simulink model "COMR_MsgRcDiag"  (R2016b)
settings: Solver=FixedStepDiscrete  StartTime=0.0  StopTime=10.0  FixedStep=0.02  RelTol=1e-3  EnableMultiTasking=on
libraries: simulink x39

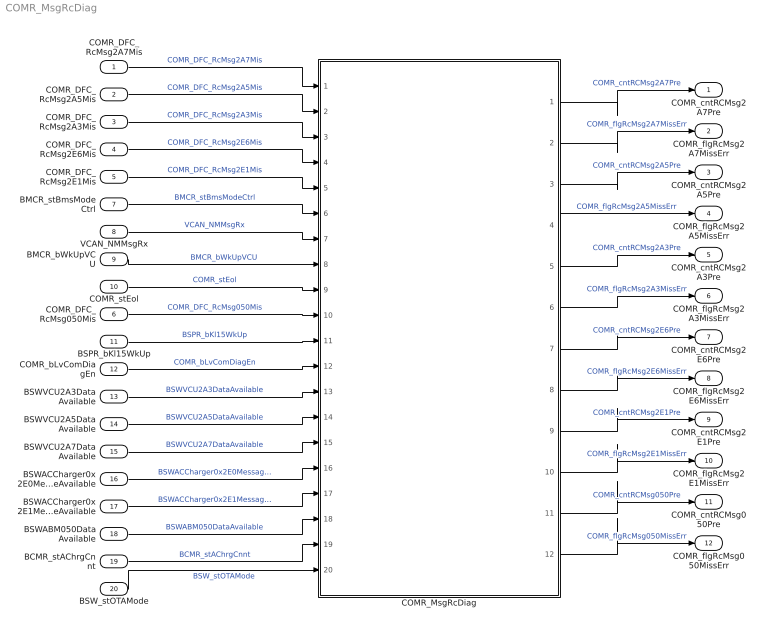
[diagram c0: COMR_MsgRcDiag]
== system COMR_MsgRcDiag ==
  COMR_DFC_RcMsg2A7Mis : Inport
  COMR_DFC_RcMsg2A5Mis : Inport  Port=2
  COMR_DFC_RcMsg2A3Mis : Inport  Port=3
  COMR_DFC_RcMsg2E6Mis : Inport  Port=4
  COMR_DFC_RcMsg2E1Mis : Inport  Port=5
  COMR_DFC_RcMsg050Mis : Inport  Port=6
  BMCR_stBmsModeCtrl : Inport  Port=7  OutDataTypeStr=uint8
  VCAN_NMMsgRx : Inport  Port=8  OutDataTypeStr=boolean
  BMCR_bWkUpVCU : Inport  Port=9  OutDataTypeStr=boolean
  COMR_stEol : Inport  Port=10  OutDataTypeStr=boolean
  BSPR_bKl15WkUp : Inport  Port=11
  COMR_bLvComDiagEn : Inport  Port=12  OutDataTypeStr=boolean
  BSWVCU2A3DataAvailable : Inport  Port=13  OutDataTypeStr=boolean
  BSWVCU2A5DataAvailable : Inport  Port=14  OutDataTypeStr=boolean
  BSWVCU2A7DataAvailable : Inport  Port=15  OutDataTypeStr=boolean
  BSWACCharger0x2E0MessageAvailable : Inport  Port=16
  BSWACCharger0x2E1MessageAvailable : Inport  Port=17  OutDataTypeStr=boolean
  BSWABM050DataAvailable : Inport  Port=18  OutDataTypeStr=boolean
  BCMR_stAChrgCnnt : Inport  Port=19
  BSW_stOTAMode : Inport  Port=20  OutDataTypeStr=boolean
  COMR_MsgRcDiag : Subsystem
  COMR_cntRCMsg2A7Pre : Outport
  COMR_flgRcMsg2A7MissErr : Outport  Port=2
  COMR_cntRCMsg2A5Pre : Outport  Port=3
  COMR_flgRcMsg2A5MissErr : Outport  Port=4
  COMR_cntRCMsg2A3Pre : Outport  Port=5
  COMR_flgRcMsg2A3MissErr : Outport  Port=6
  COMR_cntRCMsg2E6Pre : Outport  Port=7
  COMR_flgRcMsg2E6MissErr : Outport  Port=8
  COMR_cntRCMsg2E1Pre : Outport  Port=9
  COMR_flgRcMsg2E1MissErr : Outport  Port=10
  COMR_cntRCMsg050Pre : Outport  Port=11
  COMR_flgRcMsg050MissErr : Outport  Port=12
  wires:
  COMR_DFC_RcMsg2A7Mis/1 -> COMR_MsgRcDiag/1("COMR_DFC_RcMsg2A7Mis ")  "COMR_DFC_RcMsg2A7Mis"
  COMR_DFC_RcMsg2A5Mis/1 -> COMR_MsgRcDiag/2(COMR_DFC_RcMsg2A5Mis)  "COMR_DFC_RcMsg2A5Mis"
  COMR_DFC_RcMsg2A3Mis/1 -> COMR_MsgRcDiag/3(COMR_DFC_RcMsg2A3Mis)  "COMR_DFC_RcMsg2A3Mis"
  COMR_DFC_RcMsg2E6Mis/1 -> COMR_MsgRcDiag/4(COMR_DFC_RcMsg2E6Mis)  "COMR_DFC_RcMsg2E6Mis"
  COMR_DFC_RcMsg2E1Mis/1 -> COMR_MsgRcDiag/5(COMR_DFC_RcMsg2E1Mis)  "COMR_DFC_RcMsg2E1Mis"
  COMR_DFC_RcMsg050Mis/1 -> COMR_MsgRcDiag/10(COMR_DFC_RcMsg050Mis)  "COMR_DFC_RcMsg050Mis"
  COMR_MsgRcDiag/1(COMR_cntRCMsg2A7Pre) -> COMR_cntRCMsg2A7Pre/1  "COMR_cntRCMsg2A7Pre"
  COMR_MsgRcDiag/2(COMR_flgRcMsg2A7MissErr) -> COMR_flgRcMsg2A7MissErr/1  "COMR_flgRcMsg2A7MissErr"
  COMR_MsgRcDiag/3(COMR_cntRCMsg2A5Pre) -> COMR_cntRCMsg2A5Pre/1  "COMR_cntRCMsg2A5Pre"
  COMR_MsgRcDiag/4(COMR_flgRcMsg2A5MissErr) -> COMR_flgRcMsg2A5MissErr/1  "COMR_flgRcMsg2A5MissErr"
  COMR_MsgRcDiag/5(COMR_cntRCMsg2A3Pre) -> COMR_cntRCMsg2A3Pre/1  "COMR_cntRCMsg2A3Pre"
  COMR_MsgRcDiag/6(COMR_flgRcMsg2A3MissErr) -> COMR_flgRcMsg2A3MissErr/1  "COMR_flgRcMsg2A3MissErr"
  COMR_MsgRcDiag/7(COMR_cntRCMsg2E6Pre) -> COMR_cntRCMsg2E6Pre/1  "COMR_cntRCMsg2E6Pre"
  COMR_MsgRcDiag/8(COMR_flgRcMsg2E6MissErr) -> COMR_flgRcMsg2E6MissErr/1  "COMR_flgRcMsg2E6MissErr"
  COMR_MsgRcDiag/9(COMR_cntRCMsg2E1Pre) -> COMR_cntRCMsg2E1Pre/1  "COMR_cntRCMsg2E1Pre"
  COMR_MsgRcDiag/10(COMR_flgRcMsg2E1MissErr) -> COMR_flgRcMsg2E1MissErr/1  "COMR_flgRcMsg2E1MissErr"
  COMR_MsgRcDiag/12(COMR_flgRcMsg050MissErr) -> COMR_flgRcMsg050MissErr/1  "COMR_flgRcMsg050MissErr"
  BMCR_stBmsModeCtrl/1 -> COMR_MsgRcDiag/6(BMCR_stBmsModeCtrl)  "BMCR_stBmsModeCtrl"
  COMR_MsgRcDiag/11(COMR_cntRCMsg050Pre) -> COMR_cntRCMsg050Pre/1  "COMR_cntRCMsg050Pre"
  VCAN_NMMsgRx/1 -> COMR_MsgRcDiag/7(VCAN_NMMsgRx)  "VCAN_NMMsgRx"
  BMCR_bWkUpVCU/1 -> COMR_MsgRcDiag/8(BMCR_bWkUpVCU)  "BMCR_bWkUpVCU"
  COMR_stEol/1 -> COMR_MsgRcDiag/9(COMR_stEol)  "COMR_stEol"
  BSPR_bKl15WkUp/1 -> COMR_MsgRcDiag/11(BSPR_bKl15WkUp)  "BSPR_bKl15WkUp"
  COMR_bLvComDiagEn/1 -> COMR_MsgRcDiag/12(COMR_bLvComDiagEn)  "COMR_bLvComDiagEn"
  BSWVCU2A3DataAvailable/1 -> COMR_MsgRcDiag/13(BSWVCU2A3DataAvailable)  "BSWVCU2A3DataAvailable"
  BSWVCU2A5DataAvailable/1 -> COMR_MsgRcDiag/14(BSWVCU2A5DataAvailable)  "BSWVCU2A5DataAvailable"
  BSWVCU2A7DataAvailable/1 -> COMR_MsgRcDiag/15(BSWVCU2A7DataAvailable)  "BSWVCU2A7DataAvailable"
  BSWACCharger0x2E0MessageAvailable/1 -> COMR_MsgRcDiag/16(BSWACCharger0x2E0MessageAvailable)  "BSWACCharger0x2E0MessageAvailable"
  BSWACCharger0x2E1MessageAvailable/1 -> COMR_MsgRcDiag/17(BSWACCharger0x2E1MessageAvailable)  "BSWACCharger0x2E1MessageAvailable"
  BSWABM050DataAvailable/1 -> COMR_MsgRcDiag/18(BSWABM050DataAvailable)  "BSWABM050DataAvailable"
  BCMR_stAChrgCnnt/1 -> COMR_MsgRcDiag/19(BCMR_stAChrgCnnt)  "BCMR_stAChrgCnnt"
  BSW_stOTAMode/1 -> COMR_MsgRcDiag/20(BSW_stOTAMode)  "BSW_stOTAMode"

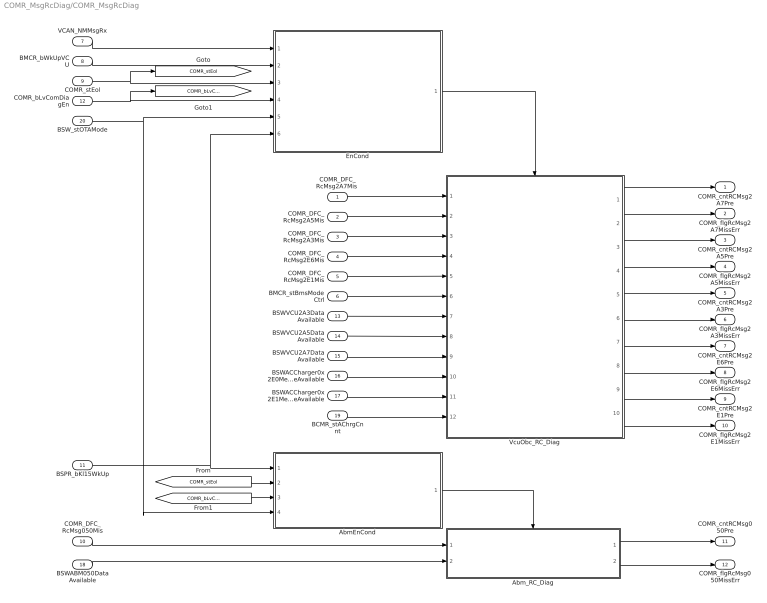
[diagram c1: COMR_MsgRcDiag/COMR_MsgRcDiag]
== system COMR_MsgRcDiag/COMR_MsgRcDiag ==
  "COMR_DFC_RcMsg2A7Mis " : Inport
  COMR_DFC_RcMsg2A5Mis : Inport  Port=2
  COMR_DFC_RcMsg2A3Mis : Inport  Port=3
  COMR_DFC_RcMsg2E6Mis : Inport  Port=4
  COMR_DFC_RcMsg2E1Mis : Inport  Port=5
  BMCR_stBmsModeCtrl : Inport  Port=6
  VCAN_NMMsgRx : Inport  Port=7  OutDataTypeStr=boolean
  BMCR_bWkUpVCU : Inport  Port=8  OutDataTypeStr=boolean
  COMR_stEol : Inport  Port=9  OutDataTypeStr=boolean
  COMR_DFC_RcMsg050Mis : Inport  Port=10
  BSPR_bKl15WkUp : Inport  Port=11  OutDataTypeStr=boolean
  COMR_bLvComDiagEn : Inport  Port=12  OutDataTypeStr=boolean
  BSWVCU2A3DataAvailable : Inport  Port=13  OutDataTypeStr=boolean
  BSWVCU2A5DataAvailable : Inport  Port=14  OutDataTypeStr=boolean
  BSWVCU2A7DataAvailable : Inport  Port=15  OutDataTypeStr=boolean
  BSWACCharger0x2E0MessageAvailable : Inport  Port=16
  BSWACCharger0x2E1MessageAvailable : Inport  Port=17  OutDataTypeStr=boolean
  BSWABM050DataAvailable : Inport  Port=18  OutDataTypeStr=boolean
  BCMR_stAChrgCnnt : Inport  Port=19
  BSW_stOTAMode : Inport  Port=20  OutDataTypeStr=boolean
  AbmEnCond : Subsystem
  Abm_RC_Diag : Subsystem
  EnCond : Subsystem
  VcuObc_RC_Diag : Subsystem
  COMR_cntRCMsg2A7Pre : Outport
  COMR_flgRcMsg2A7MissErr : Outport  Port=2
  COMR_cntRCMsg2A5Pre : Outport  Port=3
  COMR_flgRcMsg2A5MissErr : Outport  Port=4
  COMR_cntRCMsg2A3Pre : Outport  Port=5
  COMR_flgRcMsg2A3MissErr : Outport  Port=6
  COMR_cntRCMsg2E6Pre : Outport  Port=7
  COMR_flgRcMsg2E6MissErr : Outport  Port=8
  COMR_cntRCMsg2E1Pre : Outport  Port=9
  COMR_flgRcMsg2E1MissErr : Outport  Port=10
  COMR_cntRCMsg050Pre : Outport  Port=11
  COMR_flgRcMsg050MissErr : Outport  Port=12
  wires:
  VCAN_NMMsgRx/1 -> EnCond/1(VCAN_NMMsgRx)
  BMCR_bWkUpVCU/1 -> EnCond/2(BMCR_bWkUpVCU)
  COMR_stEol/1 -> EnCond/3(COMR_stEol), [COMR_stEol]
  "COMR_DFC_RcMsg2A7Mis "/1 -> VcuObc_RC_Diag/1(COMR_DFC_RcMsg2A7Mis)
  COMR_DFC_RcMsg2A5Mis/1 -> VcuObc_RC_Diag/2(COMR_DFC_RcMsg2A5Mis)
  COMR_DFC_RcMsg2A3Mis/1 -> VcuObc_RC_Diag/3(COMR_DFC_RcMsg2A3Mis)
  COMR_DFC_RcMsg2E6Mis/1 -> VcuObc_RC_Diag/4(COMR_DFC_RcMsg2E6Mis)
  COMR_DFC_RcMsg2E1Mis/1 -> VcuObc_RC_Diag/5(COMR_DFC_RcMsg2E1Mis)
  BMCR_stBmsModeCtrl/1 -> VcuObc_RC_Diag/6(BMCR_stBmsModeCtrl)
  VcuObc_RC_Diag/1(COMR_cntRCMsg2A7Pre) -> COMR_cntRCMsg2A7Pre/1
  VcuObc_RC_Diag/2(COMR_flgRcMsg2A7MissErr) -> COMR_flgRcMsg2A7MissErr/1
  VcuObc_RC_Diag/3(COMR_cntRCMsg2A5Pre) -> COMR_cntRCMsg2A5Pre/1
  VcuObc_RC_Diag/4(COMR_flgRcMsg2A5MissErr) -> COMR_flgRcMsg2A5MissErr/1
  VcuObc_RC_Diag/5(COMR_cntRCMsg2A3Pre) -> COMR_cntRCMsg2A3Pre/1
  VcuObc_RC_Diag/6(COMR_flgRcMsg2A3MissErr) -> COMR_flgRcMsg2A3MissErr/1
  VcuObc_RC_Diag/7(COMR_cntRCMsg2E6Pre) -> COMR_cntRCMsg2E6Pre/1
  VcuObc_RC_Diag/8(COMR_flgRcMsg2E6MissErr) -> COMR_flgRcMsg2E6MissErr/1
  VcuObc_RC_Diag/9(COMR_cntRCMsg2E1Pre) -> COMR_cntRCMsg2E1Pre/1
  VcuObc_RC_Diag/10(COMR_flgRcMsg2E1MissErr) -> COMR_flgRcMsg2E1MissErr/1
  EnCond/1(COMR_bMsgRcDiagEn) -> VcuObc_RC_Diag/Enable
  COMR_DFC_RcMsg050Mis/1 -> Abm_RC_Diag/1(COMR_DFC_RcMsg050Mis)
  Abm_RC_Diag/1(COMR_cntRCMsg050Pre) -> COMR_cntRCMsg050Pre/1
  Abm_RC_Diag/2(COMR_flgRcMsg050MissErr) -> COMR_flgRcMsg050MissErr/1
  AbmEnCond/1(COMR_bAbmRcDiagEn) -> Abm_RC_Diag/Enable
  BSPR_bKl15WkUp/1 -> EnCond/6(BSPR_bKl15WkUp), AbmEnCond/1(BSPR_bKl15WkUp)
  [COMR_stEol] -> AbmEnCond/2(COMR_stEol)
  COMR_bLvComDiagEn/1 -> EnCond/4(COMR_bLvComDiagEn), [COMR_bLvComDiagEn]
  [COMR_bLvComDiagEn] -> AbmEnCond/3(COMR_bLvComDiagEn)
  BSWACCharger0x2E1MessageAvailable/1 -> VcuObc_RC_Diag/11(BSWACCharger0x2E1MessageAvailable)
  BSWACCharger0x2E0MessageAvailable/1 -> VcuObc_RC_Diag/10(BSWACCharger0x2E0MessageAvailable)
  BSWVCU2A7DataAvailable/1 -> VcuObc_RC_Diag/9(BSWVCU2A7DataAvailable)
  BSWVCU2A5DataAvailable/1 -> VcuObc_RC_Diag/8(BSWVCU2A5DataAvailable)
  BSWVCU2A3DataAvailable/1 -> VcuObc_RC_Diag/7(BSWVCU2A3DataAvailable)
  BSWABM050DataAvailable/1 -> Abm_RC_Diag/2(BSWABM050DataAvailable)
  BCMR_stAChrgCnnt/1 -> VcuObc_RC_Diag/12(BCMR_stAChrgCnnt)
  BSW_stOTAMode/1 -> AbmEnCond/4(BSW_stOTAMode), EnCond/5(BSW_stOTAMode)

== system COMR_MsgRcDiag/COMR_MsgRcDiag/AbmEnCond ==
  BSPR_bKl15WkUp : Inport  OutDataTypeStr=boolean
  COMR_stEol : Inport  Port=2  OutDataTypeStr=boolean
  COMR_bLvComDiagEn : Inport  Port=3  OutDataTypeStr=boolean
  BSW_stOTAMode : Inport  Port=4  OutDataTypeStr=boolean
  Constant1 : Constant  Value=2  OutDataTypeStr=single
  Logical Operator1 : Logic  AllPortsSameDT=off  OutDataTypeStr=boolean
  Logical Operator2 : Logic  Operator=NOT  AllPortsSameDT=off  OutDataTypeStr=boolean
  Logical Operator3 : Logic  Inputs=3  AllPortsSameDT=off  OutDataTypeStr=boolean
  Logical Operator4 : Logic  Operator=NOT  AllPortsSameDT=off  OutDataTypeStr=boolean
  TONV_10msTimeDebounce : Subsystem  TreatAsAtomicUnit=on  RTWFcnName=TONV_10msTimeDebounce  RTWFileName=SrvLib
  COMR_bAbmRcDiagEn : Outport
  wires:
  Logical Operator2/1 -> Logical Operator1/2
  COMR_stEol/1 -> Logical Operator2/1
  BSPR_bKl15WkUp/1 -> Logical Operator1/1
  Logical Operator3/1 -> COMR_bAbmRcDiagEn/1  "COMR_bAbmRcDiagEn"
  Constant1/1 -> TONV_10msTimeDebounce/2(T)
  Logical Operator1/1 -> TONV_10msTimeDebounce/1(u)
  COMR_bLvComDiagEn/1 -> Logical Operator3/2
  TONV_10msTimeDebounce/1(y) -> Logical Operator3/1
  BSW_stOTAMode/1 -> Logical Operator4/1
  Logical Operator4/1 -> Logical Operator3/3

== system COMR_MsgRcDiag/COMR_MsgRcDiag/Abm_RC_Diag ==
  COMR_DFC_RcMsg050Mis : Inport
  BSWABM050DataAvailable : Inport  Port=2  OutDataTypeStr=boolean
  Enable : EnablePort  StatesWhenEnabling=reset
  Constant : Constant  Value=0  OutDataTypeStr=uint8
  DSM_ReportCheck : Subsystem  TreatAsAtomicUnit=on  RTWFcnName=DSM_ReportCheck  RTWFileName=SrvLib
  Data Store Read3 : DataStoreRead  DataStoreName=DFC_RcMsg050Mis
  Data Store Write3 : DataStoreWrite  DataStoreName=DFC_RcMsg050Mis
  Logical Operator2 : Logic  Operator=NOT  AllPortsSameDT=off  OutDataTypeStr=boolean
  Terminator : Terminator
  COMR_cntRCMsg050Pre : Outport
  COMR_flgRcMsg050MissErr : Outport  Port=2
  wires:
  COMR_DFC_RcMsg050Mis/1 -> COMR_flgRcMsg050MissErr/1, DSM_ReportCheck/2(Err), Logical Operator2/1
  DSM_ReportCheck/1(Dfc_id) -> Data Store Write3/1
  Constant/1 -> COMR_cntRCMsg050Pre/1
  Data Store Read3/1 -> DSM_ReportCheck/1(Dfc_id_nv)
  Logical Operator2/1 -> DSM_ReportCheck/3(Heal)
  BSWABM050DataAvailable/1 -> Terminator/1

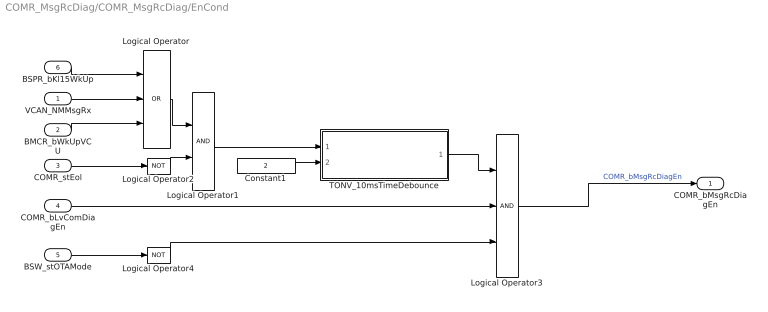
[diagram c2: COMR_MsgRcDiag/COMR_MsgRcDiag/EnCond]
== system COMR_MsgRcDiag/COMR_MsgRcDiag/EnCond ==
  VCAN_NMMsgRx : Inport  OutDataTypeStr=boolean
  BMCR_bWkUpVCU : Inport  Port=2  OutDataTypeStr=boolean
  COMR_stEol : Inport  Port=3  OutDataTypeStr=boolean
  COMR_bLvComDiagEn : Inport  Port=4  OutDataTypeStr=boolean
  BSW_stOTAMode : Inport  Port=5  OutDataTypeStr=boolean
  BSPR_bKl15WkUp : Inport  Port=6  OutDataTypeStr=boolean
  Constant1 : Constant  Value=2  OutDataTypeStr=single
  Logical Operator : Logic  Operator=OR  Inputs=3  AllPortsSameDT=off  OutDataTypeStr=boolean
  Logical Operator1 : Logic  AllPortsSameDT=off  OutDataTypeStr=boolean
  Logical Operator2 : Logic  Operator=NOT  AllPortsSameDT=off  OutDataTypeStr=boolean
  Logical Operator3 : Logic  Inputs=3  AllPortsSameDT=off  OutDataTypeStr=boolean
  Logical Operator4 : Logic  Operator=NOT  AllPortsSameDT=off  OutDataTypeStr=boolean
  TONV_10msTimeDebounce : Subsystem  TreatAsAtomicUnit=on  RTWFcnName=TONV_10msTimeDebounce  RTWFileName=SrvLib
  COMR_bMsgRcDiagEn : Outport
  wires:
  Logical Operator1/1 -> TONV_10msTimeDebounce/1(u)
  Constant1/1 -> TONV_10msTimeDebounce/2(T)
  Logical Operator3/1 -> COMR_bMsgRcDiagEn/1  "COMR_bMsgRcDiagEn"
  Logical Operator/1 -> Logical Operator1/1
  COMR_stEol/1 -> Logical Operator2/1
  Logical Operator2/1 -> Logical Operator1/2
  TONV_10msTimeDebounce/1(y) -> Logical Operator3/1
  COMR_bLvComDiagEn/1 -> Logical Operator3/2
  VCAN_NMMsgRx/1 -> Logical Operator/2
  BMCR_bWkUpVCU/1 -> Logical Operator/3
  BSPR_bKl15WkUp/1 -> Logical Operator/1
  BSW_stOTAMode/1 -> Logical Operator4/1
  Logical Operator4/1 -> Logical Operator3/3

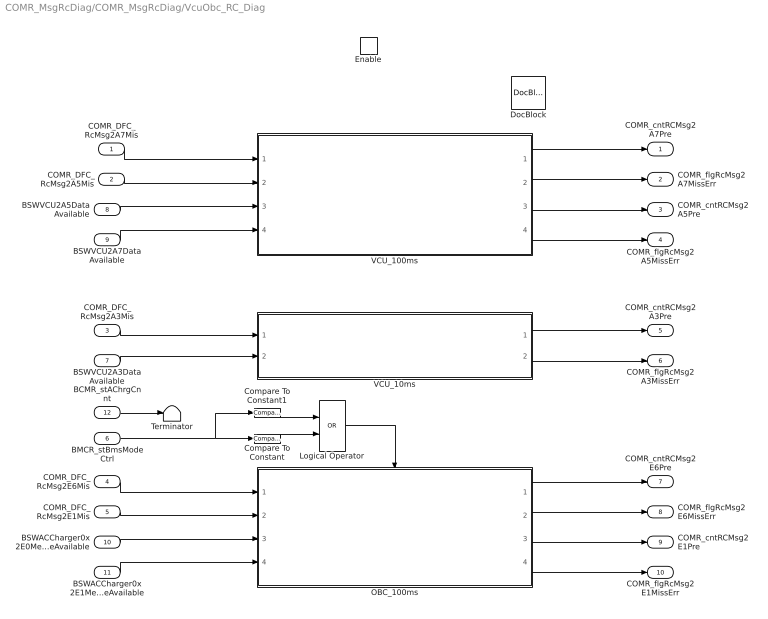
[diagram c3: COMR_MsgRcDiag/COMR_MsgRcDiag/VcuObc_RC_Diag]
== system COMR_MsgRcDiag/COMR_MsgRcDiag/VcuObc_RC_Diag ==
  COMR_DFC_RcMsg2A7Mis : Inport
  COMR_DFC_RcMsg2A5Mis : Inport  Port=2
  COMR_DFC_RcMsg2A3Mis : Inport  Port=3
  COMR_DFC_RcMsg2E6Mis : Inport  Port=4
  COMR_DFC_RcMsg2E1Mis : Inport  Port=5
  BMCR_stBmsModeCtrl : Inport  Port=6
  BSWVCU2A3DataAvailable : Inport  Port=7  OutDataTypeStr=boolean
  BSWVCU2A5DataAvailable : Inport  Port=8  OutDataTypeStr=boolean
  BSWVCU2A7DataAvailable : Inport  Port=9  OutDataTypeStr=boolean
  BSWACCharger0x2E0MessageAvailable : Inport  Port=10
  BSWACCharger0x2E1MessageAvailable : Inport  Port=11  OutDataTypeStr=boolean
  BCMR_stAChrgCnnt : Inport  Port=12
  Enable : EnablePort  StatesWhenEnabling=reset
  Compare To Constant : simulink/Logic and Bit Operations/Compare To Constant  relop===  const=6  OutDataTypeStr=boolean
  Compare To Constant1 : simulink/Logic and Bit Operations/Compare To Constant  relop===  const=11  OutDataTypeStr=boolean
  DocBlock : simulink/Model-Wide Utilities/DocBlock  DocumentType=Text
  Logical Operator : Logic  Operator=OR  AllPortsSameDT=off  OutDataTypeStr=boolean
  OBC_100ms : Subsystem
  Terminator : Terminator
  VCU_100ms : Subsystem
  VCU_10ms : Subsystem
  COMR_cntRCMsg2A7Pre : Outport  InitialOutput=[0]
  COMR_flgRcMsg2A7MissErr : Outport  Port=2  InitialOutput=[0]
  COMR_cntRCMsg2A5Pre : Outport  Port=3  InitialOutput=[0]
  COMR_flgRcMsg2A5MissErr : Outport  Port=4  InitialOutput=[0]
  COMR_cntRCMsg2A3Pre : Outport  Port=5
  COMR_flgRcMsg2A3MissErr : Outport  Port=6
  COMR_cntRCMsg2E6Pre : Outport  Port=7  InitialOutput=[0]
  COMR_flgRcMsg2E6MissErr : Outport  Port=8  InitialOutput=[0]
  COMR_cntRCMsg2E1Pre : Outport  Port=9  InitialOutput=[0]
  COMR_flgRcMsg2E1MissErr : Outport  Port=10  InitialOutput=[0]
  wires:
  COMR_DFC_RcMsg2E6Mis/1 -> OBC_100ms/1(COMR_DFC_RcMsg2E6Mis)
  COMR_DFC_RcMsg2E1Mis/1 -> OBC_100ms/2(COMR_DFC_RcMsg2E1Mis)
  OBC_100ms/1(COMR_cntRCMsg2E6Pre) -> COMR_cntRCMsg2E6Pre/1
  OBC_100ms/2(COMR_flgRcMsg2E6MissErr) -> COMR_flgRcMsg2E6MissErr/1
  OBC_100ms/3(COMR_cntRCMsg2E1Pre) -> COMR_cntRCMsg2E1Pre/1
  OBC_100ms/4(COMR_flgRcMsg2E1MissErr) -> COMR_flgRcMsg2E1MissErr/1
  BMCR_stBmsModeCtrl/1 -> Compare To Constant1/1, Compare To Constant/1
  COMR_DFC_RcMsg2A7Mis/1 -> VCU_100ms/1(COMR_DFC_RcMsg2A7Mis)
  COMR_DFC_RcMsg2A5Mis/1 -> VCU_100ms/2(COMR_DFC_RcMsg2A5Mis)
  VCU_100ms/1(COMR_cntRCMsg2A7Pre) -> COMR_cntRCMsg2A7Pre/1
  VCU_100ms/2(COMR_flgRcMsg2A7MissErr) -> COMR_flgRcMsg2A7MissErr/1
  VCU_100ms/3(COMR_cntRCMsg2A5Pre) -> COMR_cntRCMsg2A5Pre/1
  VCU_100ms/4(COMR_flgRcMsg2A5MissErr) -> COMR_flgRcMsg2A5MissErr/1
  COMR_DFC_RcMsg2A3Mis/1 -> VCU_10ms/1(COMR_DFC_RcMsg2A3Mis)
  VCU_10ms/1(COMR_cntRCMsg2A3Pre) -> COMR_cntRCMsg2A3Pre/1
  VCU_10ms/2(COMR_flgRcMsg2A3MissErr) -> COMR_flgRcMsg2A3MissErr/1
  BSWVCU2A5DataAvailable/1 -> VCU_100ms/3(BSWVCU2A5DataAvailable)
  BSWVCU2A7DataAvailable/1 -> VCU_100ms/4(BSWVCU2A7DataAvailable)
  BSWVCU2A3DataAvailable/1 -> VCU_10ms/2(BSWVCU2A3DataAvailable)
  BSWACCharger0x2E0MessageAvailable/1 -> OBC_100ms/3(BSWACCharger0x2E0MessageAvailable)
  BSWACCharger0x2E1MessageAvailable/1 -> OBC_100ms/4(BSWACCharger0x2E1MessageAvailable)
  Compare To Constant1/1 -> Logical Operator/1
  Compare To Constant/1 -> Logical Operator/2
  Logical Operator/1 -> OBC_100ms/Enable
  BCMR_stAChrgCnnt/1 -> Terminator/1

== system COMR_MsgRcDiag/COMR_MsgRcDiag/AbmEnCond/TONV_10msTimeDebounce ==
  note: Turn On Delay Time Deboune
  u : Inport
  T : Inport  Port=2
  Add : Sum
  Constant1 : Constant  Value=0  OutDataTypeStr=single
  Constant2 : Constant  OutDataTypeStr=uint8
  Constant3 : Constant  Value=0  OutDataTypeStr=uint8
  Constant4 : Constant  Value=0.01  OutDataTypeStr=single
  Delay : Delay  DelayLength=1  InitialCondition=0
  MinMax : MinMax  Inputs=2
  Product : Product  OutMin=[0]  OutMax=[65535]  OutDataTypeStr=single
  Relational Operator : RelationalOperator  Operator=>  OutDataTypeStr=boolean  RndMeth=Simplest
  Switch : Switch  Criteria=u2 ~= 0
  Switch1 : Switch  Criteria=u2 ~= 0
  y : Outport
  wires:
  Switch1/1 -> Product/1
  Constant3/1 -> Switch1/3
  Constant2/1 -> Switch1/1
  u/1 -> Switch1/2, Switch/2
  Constant4/1 -> Switch/1
  Constant1/1 -> Switch/3
  Add/1 -> Product/2
  Product/1 -> Relational Operator/1, Delay/1
  Switch/1 -> Add/1
  Delay/1 -> MinMax/2
  Relational Operator/1 -> y/1
  T/1 -> MinMax/1, Relational Operator/2
  MinMax/1 -> Add/2

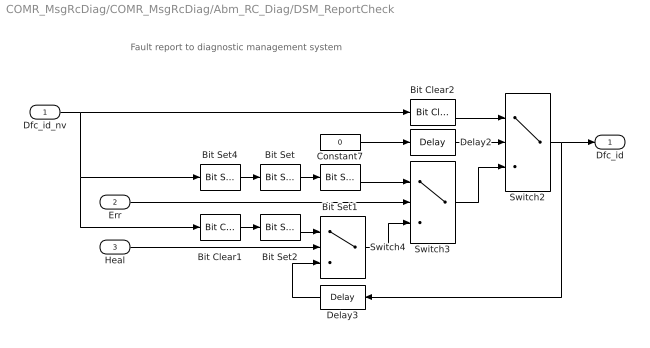
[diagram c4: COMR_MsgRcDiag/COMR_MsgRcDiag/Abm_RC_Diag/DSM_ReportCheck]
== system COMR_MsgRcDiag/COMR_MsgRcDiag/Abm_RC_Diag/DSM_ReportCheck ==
  note: Fault report to diagnostic management system
  Dfc_id_nv : Inport  OutDataTypeStr=uint8
  Err : Inport  Port=2
  Heal : Inport  Port=3
  Bit Clear1 : simulink/Logic and Bit Operations/Bit Clear  iBit=4
  Bit Clear2 : simulink/Logic and Bit Operations/Bit Clear  iBit=3
  Bit Set : simulink/Logic and Bit Operations/Bit Set  iBit=4
  Bit Set1 : simulink/Logic and Bit Operations/Bit Set  iBit=3
  Bit Set2 : simulink/Logic and Bit Operations/Bit Set  iBit=3
  Bit Set4 : simulink/Logic and Bit Operations/Bit Set  iBit=7
  Constant7 : Constant  Value=0  OutDataTypeStr=boolean
  Delay2 : Delay  DelayLength=1  InitialCondition=1
  Delay3 : Delay  DelayLength=1  InitialCondition=0
  Switch2 : Switch  Criteria=u2 ~= 0
  Switch3 : Switch  Criteria=u2 ~= 0
  Switch4 : Switch  Criteria=u2 ~= 0
  Dfc_id : Outport  OutDataTypeStr=uint8
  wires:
  Dfc_id_nv/1 -> Bit Clear2/1, Bit Set4/1, Bit Clear1/1
  Bit Set4/1 -> Bit Set/1
  Constant7/1 -> Delay2/1
  Delay2/1 -> Switch2/2
  Switch3/1 -> Switch2/3
  Bit Clear2/1 -> Switch2/1
  Switch2/1 -> Delay3/1, Dfc_id/1
  Bit Set1/1 -> Switch3/1
  Bit Set/1 -> Bit Set1/1
  Switch4/1 -> Switch3/3
  Err/1 -> Switch3/2
  Bit Set2/1 -> Switch4/1
  Bit Clear1/1 -> Bit Set2/1
  Delay3/1 -> Switch4/3
  Heal/1 -> Switch4/2

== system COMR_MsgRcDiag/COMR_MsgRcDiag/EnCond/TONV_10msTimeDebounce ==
  note: Turn On Delay Time Deboune
  u : Inport
  T : Inport  Port=2
  Add : Sum
  Constant1 : Constant  Value=0  OutDataTypeStr=single
  Constant2 : Constant  OutDataTypeStr=uint8
  Constant3 : Constant  Value=0  OutDataTypeStr=uint8
  Constant4 : Constant  Value=0.01  OutDataTypeStr=single
  Delay : Delay  DelayLength=1  InitialCondition=0
  MinMax : MinMax  Inputs=2
  Product : Product  OutMin=[0]  OutMax=[65535]  OutDataTypeStr=single
  Relational Operator : RelationalOperator  Operator=>  OutDataTypeStr=boolean  RndMeth=Simplest
  Switch : Switch  Criteria=u2 ~= 0
  Switch1 : Switch  Criteria=u2 ~= 0
  y : Outport
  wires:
  MinMax/1 -> Add/2
  T/1 -> Relational Operator/2, MinMax/1
  Relational Operator/1 -> y/1
  Delay/1 -> MinMax/2
  Switch/1 -> Add/1
  Product/1 -> Delay/1, Relational Operator/1
  Add/1 -> Product/2
  Constant1/1 -> Switch/3
  Constant4/1 -> Switch/1
  u/1 -> Switch/2, Switch1/2
  Constant2/1 -> Switch1/1
  Constant3/1 -> Switch1/3
  Switch1/1 -> Product/1

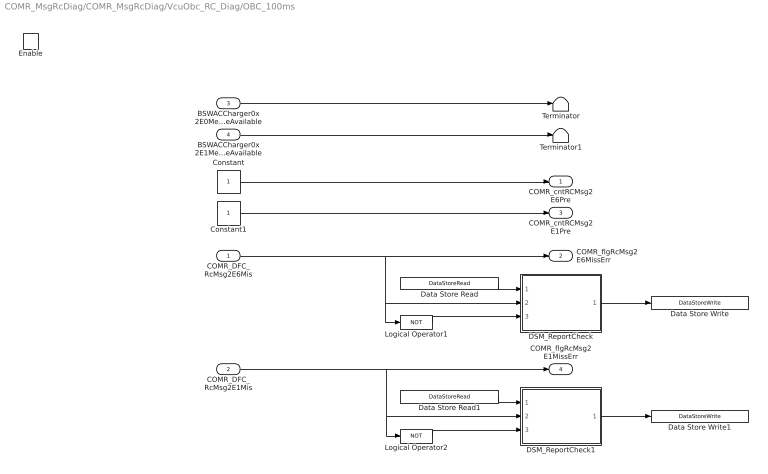
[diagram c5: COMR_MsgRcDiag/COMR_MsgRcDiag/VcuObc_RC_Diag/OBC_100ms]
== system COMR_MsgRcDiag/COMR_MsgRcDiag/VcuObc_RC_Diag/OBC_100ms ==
  COMR_DFC_RcMsg2E6Mis : Inport
  COMR_DFC_RcMsg2E1Mis : Inport  Port=2
  BSWACCharger0x2E0MessageAvailable : Inport  Port=3
  BSWACCharger0x2E1MessageAvailable : Inport  Port=4  OutDataTypeStr=boolean
  Enable : EnablePort
  Constant : Constant  OutDataTypeStr=uint8
  Constant1 : Constant  OutDataTypeStr=uint8
  DSM_ReportCheck : Subsystem  TreatAsAtomicUnit=on  RTWFcnName=DSM_ReportCheck  RTWFileName=SrvLib
  DSM_ReportCheck1 : Subsystem  TreatAsAtomicUnit=on  RTWFcnName=DSM_ReportCheck  RTWFileName=SrvLib
  Data Store Read : DataStoreRead  DataStoreName=DFC_RcMsg2E0Mis
  Data Store Read1 : DataStoreRead  DataStoreName=DFC_RcMsg2E1Mis
  Data Store Write : DataStoreWrite  DataStoreName=DFC_RcMsg2E0Mis
  Data Store Write1 : DataStoreWrite  DataStoreName=DFC_RcMsg2E1Mis
  Logical Operator1 : Logic  Operator=NOT  AllPortsSameDT=off  OutDataTypeStr=boolean
  Logical Operator2 : Logic  Operator=NOT  AllPortsSameDT=off  OutDataTypeStr=boolean
  Terminator : Terminator
  Terminator1 : Terminator
  COMR_cntRCMsg2E6Pre : Outport
  COMR_flgRcMsg2E6MissErr : Outport  Port=2  InitialOutput=[0]
  COMR_cntRCMsg2E1Pre : Outport  Port=3
  COMR_flgRcMsg2E1MissErr : Outport  Port=4  InitialOutput=[0]
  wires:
  Logical Operator1/1 -> DSM_ReportCheck/3(Heal)
  COMR_DFC_RcMsg2E6Mis/1 -> COMR_flgRcMsg2E6MissErr/1, Logical Operator1/1, DSM_ReportCheck/2(Err)
  Constant1/1 -> COMR_cntRCMsg2E1Pre/1
  Constant/1 -> COMR_cntRCMsg2E6Pre/1
  DSM_ReportCheck1/1(Dfc_id) -> Data Store Write1/1
  COMR_DFC_RcMsg2E1Mis/1 -> COMR_flgRcMsg2E1MissErr/1, Logical Operator2/1, DSM_ReportCheck1/2(Err)
  DSM_ReportCheck/1(Dfc_id) -> Data Store Write/1
  Data Store Read1/1 -> DSM_ReportCheck1/1(Dfc_id_nv)
  Data Store Read/1 -> DSM_ReportCheck/1(Dfc_id_nv)
  Logical Operator2/1 -> DSM_ReportCheck1/3(Heal)
  BSWACCharger0x2E0MessageAvailable/1 -> Terminator/1
  BSWACCharger0x2E1MessageAvailable/1 -> Terminator1/1

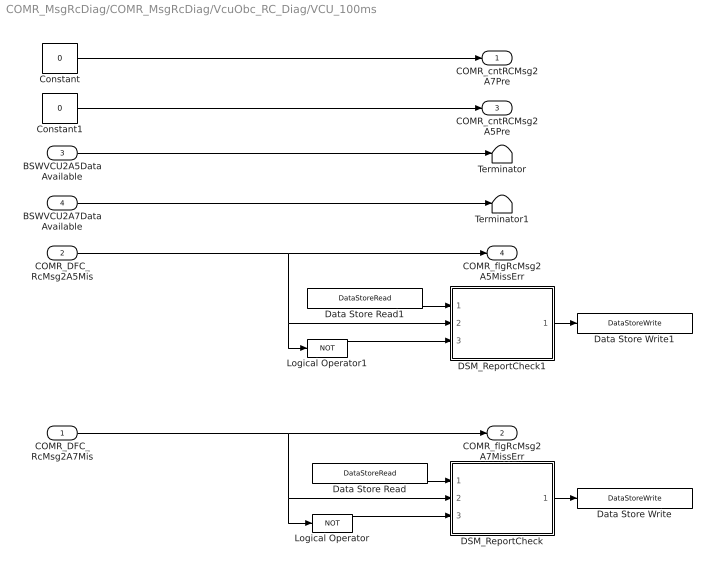
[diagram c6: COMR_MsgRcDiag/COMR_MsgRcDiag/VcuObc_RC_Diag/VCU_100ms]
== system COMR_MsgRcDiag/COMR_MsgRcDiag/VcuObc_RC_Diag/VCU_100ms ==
  COMR_DFC_RcMsg2A7Mis : Inport
  COMR_DFC_RcMsg2A5Mis : Inport  Port=2
  BSWVCU2A5DataAvailable : Inport  Port=3  OutDataTypeStr=boolean
  BSWVCU2A7DataAvailable : Inport  Port=4  OutDataTypeStr=boolean
  Constant : Constant  Value=0  OutDataTypeStr=uint8
  Constant1 : Constant  Value=0  OutDataTypeStr=uint8
  DSM_ReportCheck : Subsystem  TreatAsAtomicUnit=on  RTWFcnName=DSM_ReportCheck  RTWFileName=SrvLib
  DSM_ReportCheck1 : Subsystem  TreatAsAtomicUnit=on  RTWFcnName=DSM_ReportCheck  RTWFileName=SrvLib
  Data Store Read : DataStoreRead  DataStoreName=DFC_RcMsg2A7Mis
  Data Store Read1 : DataStoreRead  DataStoreName=DFC_RcMsg2A5Mis
  Data Store Write : DataStoreWrite  DataStoreName=DFC_RcMsg2A7Mis
  Data Store Write1 : DataStoreWrite  DataStoreName=DFC_RcMsg2A5Mis
  Logical Operator : Logic  Operator=NOT  AllPortsSameDT=off  OutDataTypeStr=boolean
  Logical Operator1 : Logic  Operator=NOT  AllPortsSameDT=off  OutDataTypeStr=boolean
  Terminator : Terminator
  Terminator1 : Terminator
  COMR_cntRCMsg2A7Pre : Outport
  COMR_flgRcMsg2A7MissErr : Outport  Port=2
  COMR_cntRCMsg2A5Pre : Outport  Port=3
  COMR_flgRcMsg2A5MissErr : Outport  Port=4
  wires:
  DSM_ReportCheck/1(Dfc_id) -> Data Store Write/1
  Logical Operator1/1 -> DSM_ReportCheck1/3(Heal)
  COMR_DFC_RcMsg2A5Mis/1 -> COMR_flgRcMsg2A5MissErr/1, DSM_ReportCheck1/2(Err), Logical Operator1/1
  Constant1/1 -> COMR_cntRCMsg2A5Pre/1
  Logical Operator/1 -> DSM_ReportCheck/3(Heal)
  Constant/1 -> COMR_cntRCMsg2A7Pre/1
  COMR_DFC_RcMsg2A7Mis/1 -> COMR_flgRcMsg2A7MissErr/1, DSM_ReportCheck/2(Err), Logical Operator/1
  Data Store Read1/1 -> DSM_ReportCheck1/1(Dfc_id_nv)
  DSM_ReportCheck1/1(Dfc_id) -> Data Store Write1/1
  Data Store Read/1 -> DSM_ReportCheck/1(Dfc_id_nv)
  BSWVCU2A5DataAvailable/1 -> Terminator/1
  BSWVCU2A7DataAvailable/1 -> Terminator1/1

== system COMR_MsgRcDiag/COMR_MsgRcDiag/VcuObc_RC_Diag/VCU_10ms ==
  COMR_DFC_RcMsg2A3Mis : Inport
  BSWVCU2A3DataAvailable : Inport  Port=2  OutDataTypeStr=boolean
  Constant : Constant  Value=0  OutDataTypeStr=uint8
  DSM_ReportCheck : Subsystem  TreatAsAtomicUnit=on  RTWFcnName=DSM_ReportCheck  RTWFileName=SrvLib
  Data Store Read2 : DataStoreRead  DataStoreName=DFC_RcMsg2A3Mis
  Data Store Write2 : DataStoreWrite  DataStoreName=DFC_RcMsg2A3Mis
  Logical Operator2 : Logic  Operator=NOT  AllPortsSameDT=off  OutDataTypeStr=boolean
  Terminator : Terminator
  COMR_cntRCMsg2A3Pre : Outport
  COMR_flgRcMsg2A3MissErr : Outport  Port=2
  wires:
  Data Store Read2/1 -> DSM_ReportCheck/1(Dfc_id_nv)
  COMR_DFC_RcMsg2A3Mis/1 -> COMR_flgRcMsg2A3MissErr/1, DSM_ReportCheck/2(Err), Logical Operator2/1
  Logical Operator2/1 -> DSM_ReportCheck/3(Heal)
  DSM_ReportCheck/1(Dfc_id) -> Data Store Write2/1
  BSWVCU2A3DataAvailable/1 -> Terminator/1
  Constant/1 -> COMR_cntRCMsg2A3Pre/1

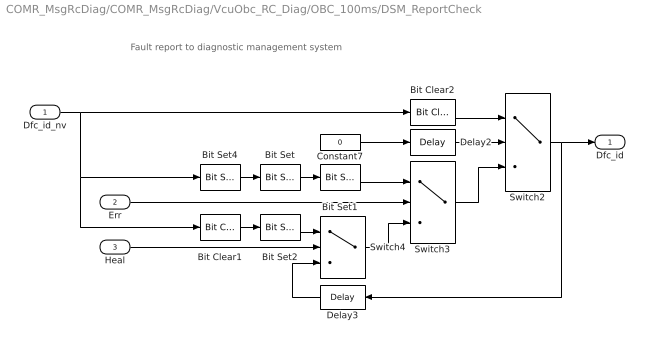
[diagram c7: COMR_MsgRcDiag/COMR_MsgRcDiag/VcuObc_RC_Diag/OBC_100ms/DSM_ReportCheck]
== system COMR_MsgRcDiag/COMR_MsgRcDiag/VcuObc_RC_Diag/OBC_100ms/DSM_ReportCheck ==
  note: Fault report to diagnostic management system
  Dfc_id_nv : Inport  OutDataTypeStr=uint8
  Err : Inport  Port=2
  Heal : Inport  Port=3
  Bit Clear1 : simulink/Logic and Bit Operations/Bit Clear  iBit=4
  Bit Clear2 : simulink/Logic and Bit Operations/Bit Clear  iBit=3
  Bit Set : simulink/Logic and Bit Operations/Bit Set  iBit=4
  Bit Set1 : simulink/Logic and Bit Operations/Bit Set  iBit=3
  Bit Set2 : simulink/Logic and Bit Operations/Bit Set  iBit=3
  Bit Set4 : simulink/Logic and Bit Operations/Bit Set  iBit=7
  Constant7 : Constant  Value=0  OutDataTypeStr=boolean
  Delay2 : Delay  DelayLength=1  InitialCondition=1
  Delay3 : Delay  DelayLength=1  InitialCondition=0
  Switch2 : Switch  Criteria=u2 ~= 0
  Switch3 : Switch  Criteria=u2 ~= 0
  Switch4 : Switch  Criteria=u2 ~= 0
  Dfc_id : Outport  OutDataTypeStr=uint8
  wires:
  Dfc_id_nv/1 -> Bit Clear2/1, Bit Set4/1, Bit Clear1/1
  Bit Set4/1 -> Bit Set/1
  Constant7/1 -> Delay2/1
  Delay2/1 -> Switch2/2
  Switch3/1 -> Switch2/3
  Bit Clear2/1 -> Switch2/1
  Switch2/1 -> Delay3/1, Dfc_id/1
  Bit Set1/1 -> Switch3/1
  Bit Set/1 -> Bit Set1/1
  Switch4/1 -> Switch3/3
  Err/1 -> Switch3/2
  Bit Set2/1 -> Switch4/1
  Bit Clear1/1 -> Bit Set2/1
  Delay3/1 -> Switch4/3
  Heal/1 -> Switch4/2

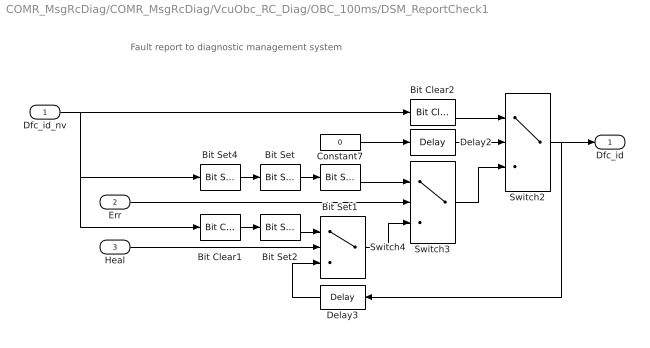
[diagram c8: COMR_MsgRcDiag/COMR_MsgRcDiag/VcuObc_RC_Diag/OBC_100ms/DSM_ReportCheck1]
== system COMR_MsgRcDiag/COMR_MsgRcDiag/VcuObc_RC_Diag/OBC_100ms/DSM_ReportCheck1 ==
  note: Fault report to diagnostic management system
  Dfc_id_nv : Inport  OutDataTypeStr=uint8
  Err : Inport  Port=2
  Heal : Inport  Port=3
  Bit Clear1 : simulink/Logic and Bit Operations/Bit Clear  iBit=4
  Bit Clear2 : simulink/Logic and Bit Operations/Bit Clear  iBit=3
  Bit Set : simulink/Logic and Bit Operations/Bit Set  iBit=4
  Bit Set1 : simulink/Logic and Bit Operations/Bit Set  iBit=3
  Bit Set2 : simulink/Logic and Bit Operations/Bit Set  iBit=3
  Bit Set4 : simulink/Logic and Bit Operations/Bit Set  iBit=7
  Constant7 : Constant  Value=0  OutDataTypeStr=boolean
  Delay2 : Delay  DelayLength=1  InitialCondition=1
  Delay3 : Delay  DelayLength=1  InitialCondition=0
  Switch2 : Switch  Criteria=u2 ~= 0
  Switch3 : Switch  Criteria=u2 ~= 0
  Switch4 : Switch  Criteria=u2 ~= 0
  Dfc_id : Outport  OutDataTypeStr=uint8
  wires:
  Dfc_id_nv/1 -> Bit Clear2/1, Bit Set4/1, Bit Clear1/1
  Bit Set4/1 -> Bit Set/1
  Constant7/1 -> Delay2/1
  Delay2/1 -> Switch2/2
  Switch3/1 -> Switch2/3
  Bit Clear2/1 -> Switch2/1
  Switch2/1 -> Delay3/1, Dfc_id/1
  Bit Set1/1 -> Switch3/1
  Bit Set/1 -> Bit Set1/1
  Switch4/1 -> Switch3/3
  Err/1 -> Switch3/2
  Bit Set2/1 -> Switch4/1
  Bit Clear1/1 -> Bit Set2/1
  Delay3/1 -> Switch4/3
  Heal/1 -> Switch4/2

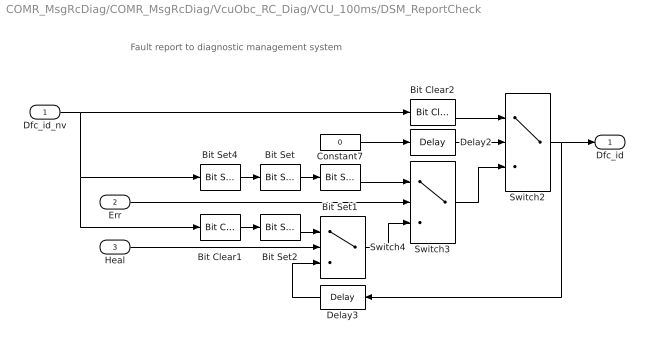
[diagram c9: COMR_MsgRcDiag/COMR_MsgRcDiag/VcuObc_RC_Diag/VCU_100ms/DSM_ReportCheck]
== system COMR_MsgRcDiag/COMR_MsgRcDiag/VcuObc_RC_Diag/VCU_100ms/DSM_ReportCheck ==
  note: Fault report to diagnostic management system
  Dfc_id_nv : Inport  OutDataTypeStr=uint8
  Err : Inport  Port=2
  Heal : Inport  Port=3
  Bit Clear1 : simulink/Logic and Bit Operations/Bit Clear  iBit=4
  Bit Clear2 : simulink/Logic and Bit Operations/Bit Clear  iBit=3
  Bit Set : simulink/Logic and Bit Operations/Bit Set  iBit=4
  Bit Set1 : simulink/Logic and Bit Operations/Bit Set  iBit=3
  Bit Set2 : simulink/Logic and Bit Operations/Bit Set  iBit=3
  Bit Set4 : simulink/Logic and Bit Operations/Bit Set  iBit=7
  Constant7 : Constant  Value=0  OutDataTypeStr=boolean
  Delay2 : Delay  DelayLength=1  InitialCondition=1
  Delay3 : Delay  DelayLength=1  InitialCondition=0
  Switch2 : Switch  Criteria=u2 ~= 0
  Switch3 : Switch  Criteria=u2 ~= 0
  Switch4 : Switch  Criteria=u2 ~= 0
  Dfc_id : Outport  OutDataTypeStr=uint8
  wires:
  Dfc_id_nv/1 -> Bit Clear2/1, Bit Set4/1, Bit Clear1/1
  Bit Set4/1 -> Bit Set/1
  Constant7/1 -> Delay2/1
  Delay2/1 -> Switch2/2
  Switch3/1 -> Switch2/3
  Bit Clear2/1 -> Switch2/1
  Switch2/1 -> Delay3/1, Dfc_id/1
  Bit Set1/1 -> Switch3/1
  Bit Set/1 -> Bit Set1/1
  Switch4/1 -> Switch3/3
  Err/1 -> Switch3/2
  Bit Set2/1 -> Switch4/1
  Bit Clear1/1 -> Bit Set2/1
  Delay3/1 -> Switch4/3
  Heal/1 -> Switch4/2

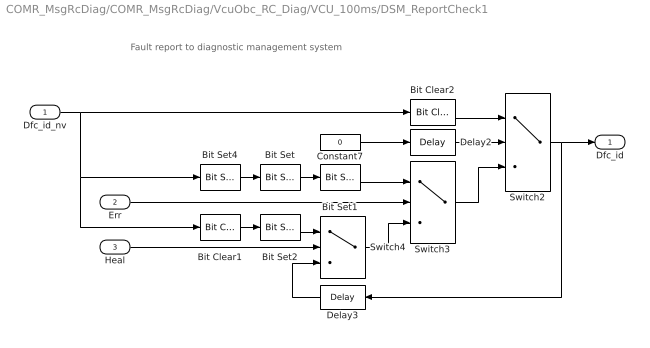
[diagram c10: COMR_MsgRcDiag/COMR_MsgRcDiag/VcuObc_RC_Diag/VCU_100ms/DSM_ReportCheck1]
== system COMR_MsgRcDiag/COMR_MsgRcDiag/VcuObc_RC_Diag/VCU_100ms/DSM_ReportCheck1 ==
  note: Fault report to diagnostic management system
  Dfc_id_nv : Inport  OutDataTypeStr=uint8
  Err : Inport  Port=2
  Heal : Inport  Port=3
  Bit Clear1 : simulink/Logic and Bit Operations/Bit Clear  iBit=4
  Bit Clear2 : simulink/Logic and Bit Operations/Bit Clear  iBit=3
  Bit Set : simulink/Logic and Bit Operations/Bit Set  iBit=4
  Bit Set1 : simulink/Logic and Bit Operations/Bit Set  iBit=3
  Bit Set2 : simulink/Logic and Bit Operations/Bit Set  iBit=3
  Bit Set4 : simulink/Logic and Bit Operations/Bit Set  iBit=7
  Constant7 : Constant  Value=0  OutDataTypeStr=boolean
  Delay2 : Delay  DelayLength=1  InitialCondition=1
  Delay3 : Delay  DelayLength=1  InitialCondition=0
  Switch2 : Switch  Criteria=u2 ~= 0
  Switch3 : Switch  Criteria=u2 ~= 0
  Switch4 : Switch  Criteria=u2 ~= 0
  Dfc_id : Outport  OutDataTypeStr=uint8
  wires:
  Heal/1 -> Switch4/2
  Delay3/1 -> Switch4/3
  Bit Clear1/1 -> Bit Set2/1
  Bit Set2/1 -> Switch4/1
  Err/1 -> Switch3/2
  Switch4/1 -> Switch3/3
  Bit Set/1 -> Bit Set1/1
  Bit Set1/1 -> Switch3/1
  Switch2/1 -> Dfc_id/1, Delay3/1
  Bit Clear2/1 -> Switch2/1
  Switch3/1 -> Switch2/3
  Delay2/1 -> Switch2/2
  Constant7/1 -> Delay2/1
  Bit Set4/1 -> Bit Set/1
  Dfc_id_nv/1 -> Bit Clear1/1, Bit Set4/1, Bit Clear2/1

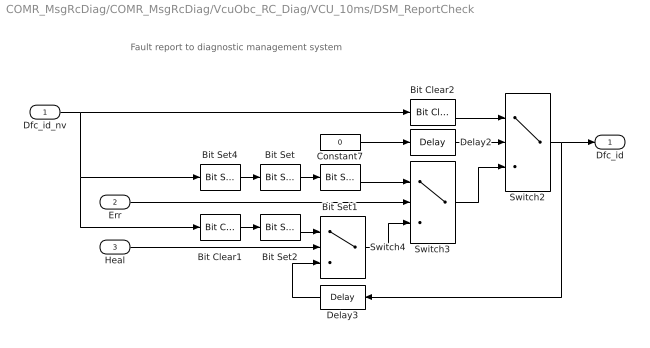
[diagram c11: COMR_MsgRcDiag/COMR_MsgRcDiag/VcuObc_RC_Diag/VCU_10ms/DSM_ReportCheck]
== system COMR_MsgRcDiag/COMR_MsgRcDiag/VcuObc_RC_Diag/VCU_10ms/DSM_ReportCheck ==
  note: Fault report to diagnostic management system
  Dfc_id_nv : Inport  OutDataTypeStr=uint8
  Err : Inport  Port=2
  Heal : Inport  Port=3
  Bit Clear1 : simulink/Logic and Bit Operations/Bit Clear  iBit=4
  Bit Clear2 : simulink/Logic and Bit Operations/Bit Clear  iBit=3
  Bit Set : simulink/Logic and Bit Operations/Bit Set  iBit=4
  Bit Set1 : simulink/Logic and Bit Operations/Bit Set  iBit=3
  Bit Set2 : simulink/Logic and Bit Operations/Bit Set  iBit=3
  Bit Set4 : simulink/Logic and Bit Operations/Bit Set  iBit=7
  Constant7 : Constant  Value=0  OutDataTypeStr=boolean
  Delay2 : Delay  DelayLength=1  InitialCondition=1
  Delay3 : Delay  DelayLength=1  InitialCondition=0
  Switch2 : Switch  Criteria=u2 ~= 0
  Switch3 : Switch  Criteria=u2 ~= 0
  Switch4 : Switch  Criteria=u2 ~= 0
  Dfc_id : Outport  OutDataTypeStr=uint8
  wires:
  Dfc_id_nv/1 -> Bit Clear2/1, Bit Set4/1, Bit Clear1/1
  Bit Set4/1 -> Bit Set/1
  Constant7/1 -> Delay2/1
  Delay2/1 -> Switch2/2
  Switch3/1 -> Switch2/3
  Bit Clear2/1 -> Switch2/1
  Switch2/1 -> Delay3/1, Dfc_id/1
  Bit Set1/1 -> Switch3/1
  Bit Set/1 -> Bit Set1/1
  Switch4/1 -> Switch3/3
  Err/1 -> Switch3/2
  Bit Set2/1 -> Switch4/1
  Bit Clear1/1 -> Bit Set2/1
  Delay3/1 -> Switch4/3
  Heal/1 -> Switch4/2
